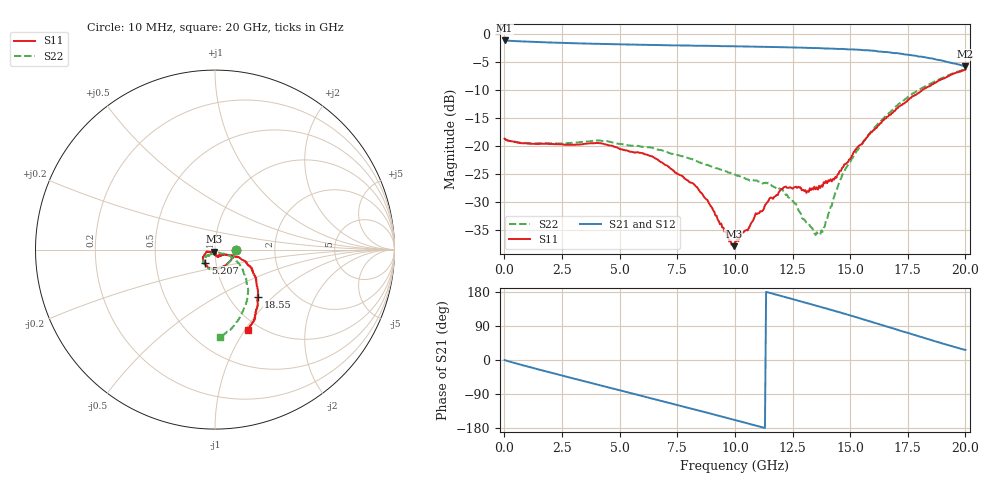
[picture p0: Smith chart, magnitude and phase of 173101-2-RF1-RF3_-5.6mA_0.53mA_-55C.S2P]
!  2-Port S-parameters saved by WinCal
! VAR MeasName=S-Parameters (CALIBRATED_DATA) read from VNA (N5242A)
! VAR MeasDate=2017-7-20 10:26:57
! VAR NAME=173101-2-RF1-RF3_-5.6mA_0.53mA_-55C
! VAR FILENAME=173101-2-RF1-RF3_-5.6mA_0.53mA_-55C.S2P
! VAR DATE=2017-7-20 10:26:57
! VAR PHYS_PORTS=1,2
# Hz S DB R 50
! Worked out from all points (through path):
!   401 points, 10 MHz to 20 GHz, reference 50 ohm
!   highest |S21| = -1.13 dB at 10 MHz (marker M1); lowest = -5.7 dB at 20 GHz (marker M2)
!   group delay of S21, straight-line fit = 45.8 ps
!   lowest |S11| = -37.8 dB at 9.955 GHz (marker M3), VSWR 1.03, Z = 49.5 - j1.19 ohm
!   |S11| at or under -10 dB: start of sweep to 18.12 GHz
!   |S22| runs from -35.8 to -6.2 dB; largest |S21 - S12| = 0.0091
!   S11 on the Smith chart (normalised r, x): 10 MHz: 1.26, -0.01; 5.207 GHz: 0.89, -0.13; 18.55 GHz: 1.35, -0.81; 20 GHz: 0.88, -1.03
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1e7  -18.64 -2.3  -1.13 -0.1  -1.13 -0.1  -18.61 -2.1
1.6092e9  -19.54 -52.8  -1.44 -26.9  -1.45 -26.9  -19.44 -51.2
3.358325e9  -19.64 -94.4  -1.66 -54.4  -1.67 -54.4  -19.20 -89.9
4.157925e9  -19.45 -110.7  -1.75 -66.8  -1.76 -66.8  -18.97 -105.5
5.2074e9  -20.67 -125.9  -1.85 -83.1  -1.87 -83.0  -19.67 -117.2
6.70665e9  -22.58 -148.9  -1.95 -106.4  -1.95 -106.3  -20.63 -135.7
8.30585e9  -27.14 -165.0  -2.07 -131.3  -2.08 -131.3  -22.55 -145.8
9.855075e9  -37.55 -116.1  -2.16 -156.0  -2.17 -156.1  -24.79 -144.7
9.955025e9  -37.80 -110.9  -2.16 -157.6  -2.19 -157.7  -24.93 -144.3
1.0005e10  -37.08 -111.8  -2.18 -158.4  -2.20 -158.5  -25.03 -144.3
1.145428e10  -29.74 -80.2  -2.28 178.1  -2.30 178.2  -26.48 -131.7
1.210395e10  -27.38 -66.4  -2.34 167.4  -2.35 167.5  -28.01 -133.9
1.335332e10  -27.47 -50.8  -2.47 146.3  -2.45 146.3  -34.60 -91.5
1.355322e10  -27.32 -45.6  -2.48 142.9  -2.49 142.7  -35.33 -77.8
1.375312e10  -26.97 -45.2  -2.52 139.4  -2.52 139.4  -34.97 -67.7
1.430285e10  -25.94 -33.4  -2.61 129.9  -2.62 129.9  -29.05 -33.6
1.475262e10  -23.20 -24.2  -2.66 122.0  -2.67 121.8  -24.35 -23.5
1.590205e10  -17.55 -18.7  -2.93 101.0  -2.94 100.7  -17.37 -28.2
1.670165e10  -14.40 -22.2  -3.24 86.3  -3.32 85.9  -14.01 -37.6
1.76012e10  -11.41 -33.3  -3.73 69.8  -3.73 69.7  -10.89 -49.8
1.855072e10  -8.99 -47.8  -4.33 51.9  -4.43 52.0  -8.70 -64.0
2e10  -6.31 -67.9  -5.71 26.6  -5.78 27.2  -6.22 -86.6
